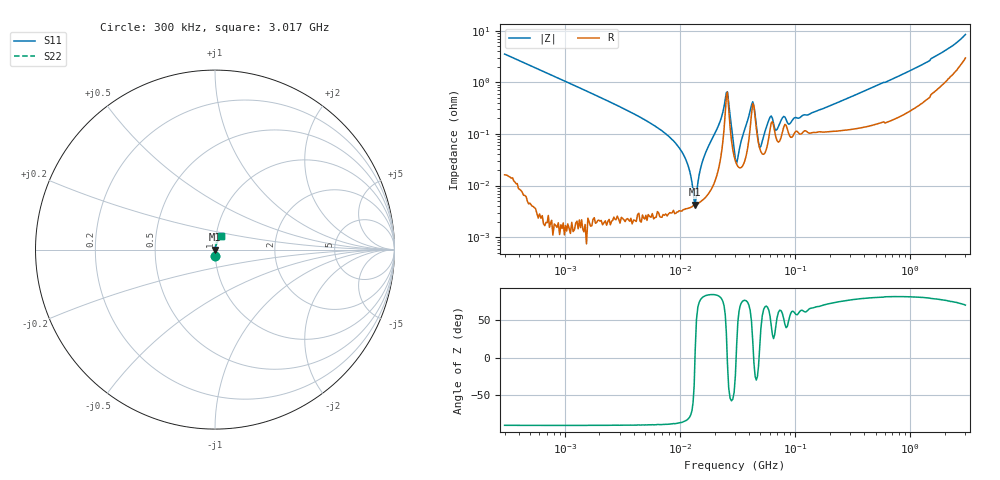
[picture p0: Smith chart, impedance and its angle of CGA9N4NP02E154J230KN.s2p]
! S-Parameter Data Generated by TDK Corporation
! Copyright(C) 2024 TDK Corporation.
! All Rights Reserved.
! TDK P/N: CGA9N4NP02E154J230KN (Multilayer Ceramic Chip Capacitor)
! Property: C=150nF
! Size(LxWxT): 5.7x5x2.3mm
! Model Type: s2p (Touchstone File Format Version 1.0)
! Frequency: DC=Yes Start=0.3MHz Stop=3016.958361MHz 374points Log-sweep
! Model Generated on May 28, 2024
! Terms and conditions regarding TDK Simulation Models:
! 1)This simulation model is being provided solely for informational
!  purposes. Please refer to the specifications of the products in
!  terms of detailed characteristics of such products.
! 2)In no event shall TDK Corporation of any of its subsidiaries be
!  liable for any loss or damage arising, directly or indirectly,
!  from any information contained in this simulation model, including,
!  but not limited to loss or damages arising from any inaccuracies,
!  omissions or errors in connection with such information.
! 3)Any and all copyrights on this simulation model are owned by
!  TDK Corporation.  Duplication or redistribution of this simulation
!  model without prior written permission from TDK Corporation
!  is prohibited.
! 4)This simulation model is subject to any modification or change
!  without any prior notice.
! 5)Neither TDK Corporation nor any of its subsidiaries shall make any
!  warranty, express or implied, including but not limited to the
!  correctness, implied warranties of merchantability and fitness for
!  a particular purpose with respect to this simulation models.
! 6)The use of this simulation model shall be deemed to have consented
!  to the terms and conditions hereof.
! Port Assignments:
!  1 ---| |--- 2
! Applicable Conditions:
!  Temperature = 25 degC
!  DC Bias Voltage = 0 V
!  Small Signal Operation
# Hz S MA R 50
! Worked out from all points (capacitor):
!   373 points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, 300 kHz to 3.017 GHz, reference 50 ohm
!   read as one part in series: C = 150 nF near 308.6 kHz
!   lowest |Z| = 4.26 mohm at 13.58 MHz (marker M1)
!   series resonance near 13.52 MHz, so ESL is about 920 pH
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300000  0.03525 -87.7  0.9992 2.0  0.9992 2.0  0.03525 -87.7
1400461  0.007485 -89.4  1 0.4  1 0.4  0.007485 -89.4
6524543  0.001275 -88.6  1 0.1  1 0.1  0.001275 -88.6
1.038318e7  0.000452 -85.9  1 0.0  1 0.0  0.000452 -85.9
1.300178e7  8.081e-05 -59.9  1 0.0  1 0.0  8.081e-05 -59.9
1.358369e7  4.259e-05 11.1  1 -0.0  1 -0.0  4.259e-05 11.1
1.432563e7  0.0001146 67.3  1 -0.0  1 -0.0  0.0001146 67.3
1.633279e7  0.0003799 81.4  0.9999 -0.0  0.9999 -0.0  0.0003799 81.4
2.253428e7  0.001854 79.6  0.9997 -0.1  0.9997 -0.1  0.001854 79.6
2.530354e7  0.006333 32.6  0.9947 -0.2  0.9947 -0.2  0.006333 32.6
2.585739e7  0.006472 -7.0  0.9936 0.0  0.9936 0.0  0.006472 -7.0
3.032632e7  0.0003255 -23.4  0.9997 0.0  0.9997 0.0  0.0003255 -23.4
3.109046e7  0.0002694 16.4  0.9997 -0.0  0.9997 -0.0  0.0002694 16.4
4.28954e7  0.004177 22.1  0.9961 -0.1  0.9961 -0.1  0.004177 22.1
4.922114e7  0.0005457 11.9  0.9995 -0.0  0.9995 -0.0  0.0005457 11.9
6.209182e7  0.002223 42.9  0.9984 -0.1  0.9984 -0.1  0.002223 42.9
6.791023e7  0.001174 40.7  0.9991 -0.0  0.9991 -0.0  0.001174 40.7
7.964712e7  0.00218 51.6  0.9986 -0.1  0.9986 -0.1  0.00218 51.6
8.767476e7  0.001549 47.5  0.999 -0.1  0.999 -0.1  0.001549 47.5
1.401524e8  0.002561 65.5  0.9989 -0.1  0.9989 -0.1  0.002561 65.5
6.649102e8  0.01094 80.1  0.9982 -0.6  0.9982 -0.6  0.01094 80.1
3.016958e9  0.08171 65.1  0.9684 -4.4  0.9684 -4.4  0.08171 65.1
